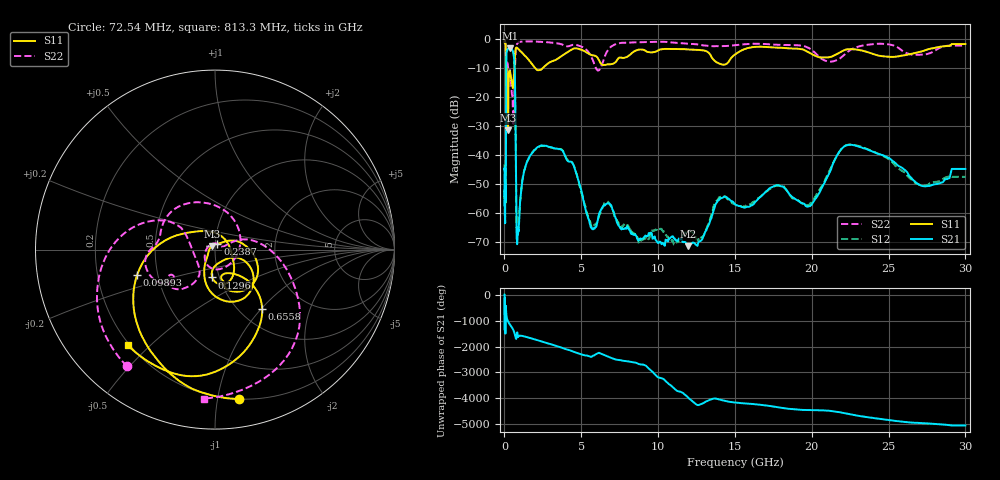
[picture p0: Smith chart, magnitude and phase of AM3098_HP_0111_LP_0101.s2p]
! Date/Time: Thu, Feb 28, 2019 8:38 AM
! Network Analyzer: Agilent Technologies E8364B Rev: A.07.50.67
! Sweep from 0.010 to 30.000 GHz, 1601 Points, Sweep Type: LOG
! Power Supply: 5.022 V, 0.002 A
# Hz S DB R 50
!freq MagS11 AngS11 MagS21 AngS21 MagS12 AngS12 MagS22 AngS22
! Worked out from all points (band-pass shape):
!   1601 points, 10 MHz to 30 GHz, reference 50 ohm
!   highest |S21| = -3.10 dB at 387.8 MHz (marker M1); lowest = -71.5 dB at 11.95 GHz (marker M2)
!   |S21| within 3 dB of the highest: 121 MHz to 619.1 MHz (498.1 MHz wide, 135 % of centre)
!   lowest |S11| = -31.4 dB at 231.6 MHz (marker M3), VSWR 1.06, Z = 48.3 + j2.01 ohm
!   |S11| at or under -10 dB: 102.2 MHz to 632.3 MHz (530.1 MHz wide, 144 % of centre); 2.022 GHz to 2.461 GHz (439 MHz wide, 19.6 % of centre)
!   |S22| runs from -29.2 to -0.5 dB; largest |S21 - S12| = 0.011
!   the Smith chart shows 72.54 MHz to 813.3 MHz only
!   S11 on the Smith chart (normalised r, x): 72.54 MHz: 0.20, -1.15; 98.93 MHz: 0.38, -0.13; 129.6 MHz: 0.92, -0.29; 238.7 MHz: 1.02, +0.07; 655.8 MHz: 1.26, -1.02; 813.3 MHz: 0.19, -0.43
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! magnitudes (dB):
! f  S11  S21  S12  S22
! 10 MHz  -0.3  -45.0  -43.1  -0.5
! 38.04 MHz  -0.5  -62.1  -59.4  -0.8
! 72.54 MHz  -1.5  -51.9  -52.2  -1.8
! 84.29 MHz  -2.4  -53.4  -53.5  -2.6
! 98.93 MHz  -6.8  -26.2  -26.1  -7.8
! 129.6 MHz  -16.2  -5.1  -5.1  -10.0
! 144.7 MHz  -20.1  -4.1  -4.1  -11.2
! 184.9 MHz  -10.7  -3.7  -3.7  -8.0
! 231.6 MHz  -31.4  -3.2  -3.2  -9.6
! 238.7 MHz  -29.1  -3.2  -3.2  -9.7
! 387.8 MHz  -12.0  -3.1  -3.1  -12.3
! 550.5 MHz  -16.8  -4.1  -4.1  -24.9
! 655.8 MHz  -7.5  -9.1  -9.1  -16.4
! 813.3 MHz  -2.8  -68.9  -67.6  -1.6
! 2.084 GHz  -10.4  -37.6  -37.8  -0.7
! 3.742 GHz  -5.6  -38.3  -38.2  -1.7
! 5.697 GHz  -5.5  -65.5  -64.9  -6.5
! 7.926 GHz  -6.2  -65.5  -64.2  -1.1
! 11.95 GHz  -3.5  -71.5  -66.8  -1.4
! 19.7 GHz  -4.2  -57.9  -57.3  -2.7
! 22.67 GHz  -3.4  -36.5  -36.4  -3.2
! 30 GHz  -1.6  -44.8  -47.5  -2.2
